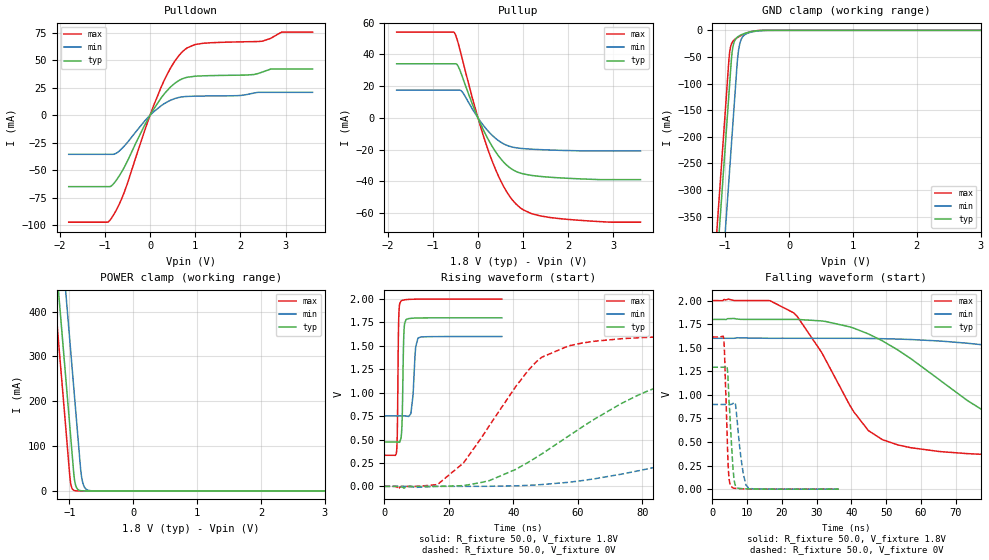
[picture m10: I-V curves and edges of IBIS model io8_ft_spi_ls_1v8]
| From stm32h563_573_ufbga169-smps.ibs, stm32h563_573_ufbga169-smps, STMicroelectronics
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[Model]   io8_ft_spi_ls_1v8
Model_type I/O
Polarity   Non-Inverting
Enable   Active-Low
| CAP_THRESHOLD on pad IOFT is "UDTCAPC" :
| Rising=20.0% of vddiom   Falling=80.0% of vddiom
| C_comp min and max val. don't necessarily correlate with the min and max pvt
| but are the smallest and greatest pad capacitance found.
| var   typ   min   max
C_comp   4.56187pF  4.45385pF  4.74999pF
|C_comp_pullup   2.85180pF  2.67180pF  2.77200pF
|C_comp_pulldown   1.71007pF  1.78205pF  1.97799pF
Vinl = 480.0mV
Vinh = 1.4V
Vmeas = 900.0mV   | Reference voltage for timing measurements
Cref  = 50.0pF   | Timing specification test load capacitance value
Rref  = 100.0MOhm   | Timing specification test load resistance value
Vref  = 900.0mV   | Timing specification test load voltage
[Model Spec]
| TIME_THRESHOLD on pin ZIV11 is "CMOS" :
| Rising=40.0% of vdd   Falling=60.0% of vdd
Vinl 703.80000mV 631.80000mV 784.80000mV
Vinh 1.06220V 937.20000mV 1.16620V
| variable   typ   min   max
[Temperature Range] 25.0 125.0 -40.0
| variable   typ   min   max
[Voltage Range] 1.8V 1.6V 2.0V
| variable   typ   min   max
[POWER Clamp Reference] 1.8V 1.6V 2.0V
| variable   typ   min   max
[GND Clamp Reference] 0V 0V 0V
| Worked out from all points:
|   slope of the pulldown table from 0 to 0.27 V, typ, clamps not added: 15.8 ohm
|   slope of the pullup table from 0 to 0.27 V, typ, clamps not added: 17.1 ohm
|   GND clamp passes 1 mA (typ) near -0.52 V on its own axis
|   POWER clamp passes 1 mA (typ) near -0.84 V on its own axis
|   rising waveform, R_fixture 50.0, V_fixture 1.8V: 20-80 % time 428ps typ, 866ps min, 322ps max; typ from 0.474 V to 1.8 V
|   falling waveform, R_fixture 50.0, V_fixture 1.8V: 20-80 % time 33.3ns typ, 83.7ns min, 16.5ns max; typ from 1.8 V to 0.474 V
|   rising waveform, R_fixture 50.0, V_fixture 0V: 20-80 % time 38.2ns typ, 81.8ns min, 20ns max; typ from 0 V to 1.29 V
|   falling waveform, R_fixture 50.0, V_fixture 0V: 20-80 % time 1.2ns typ, 1.69ns min, 842ps max; typ from 1.29 V to 0 V
[POWER Clamp]
-1.8V     1.518A     1.709A     1.407A
-1.23V    548.8mA    740.2mA    437.5mA
-1.16V    429.8mA    621.2mA    318.5mA
-1.05V    242.8mA    434.2mA    131.5mA
-980mV    123.8mA    315.2mA    17.95mA
-930mV    38.81mA    230.2mA    1.49mA
-910mV    17.82mA    196.2mA    550.8uA
-890mV    8.18mA     162.2mA    203.5uA
-810mV    363.5uA    33.6mA     3.797uA
-770mV    76.62uA    10.47mA    518.8nA
-710mV    7.417uA    1.822mA    26.38nA
3.6V      0A         0A         0A
[GND Clamp]
-1.8V     -1.581A    -1.742A    -1.516A
-1.24V    -628.8mA   -789.9mA   -564.1mA
-1.05V    -305.8mA   -466.9mA   -241.1mA
-940mV    -118.8mA   -279.9mA   -54.1mA
-930mV    -101.8mA   -262.9mA   -41.86mA
-900mV    -51.51mA   -211.9mA   -25.34mA
-880mV    -32.22mA   -177.9mA   -21mA
-810mV    -13.02mA   -59.5mA    -13.82mA
-770mV    -9.8mA     -24.99mA   -11mA
-680mV    -5.275mA   -7.288mA   -5.917mA
-400mV    -107uA     -349.1uA   -42.51uA
3.6V      5.392nA    968.2nA    261.3pA
| variable   typ   min   max
[Pullup Reference] 1.8V 1.6V 2.0V
| variable   typ   min   max
[Pulldown Reference] 0V 0V 0V
[Pullup]
-1.8V     34.12mA    17.47mA    54.1mA
-520mV    34.12mA    17.47mA    53.62mA
-450mV    33.13mA    17.47mA    48.39mA
-350mV    26.32mA    16.48mA    37.5mA
0V        9.62pA     772pA      6.41pA
300mV     -17.25mA   -10.57mA   -26.11mA
610mV     -29.08mA   -16.97mA   -45.33mA
770mV     -32.67mA   -18.47mA   -52mA
930mV     -34.74mA   -19.19mA   -56.56mA
1.18V     -36.29mA   -19.75mA   -60.37mA
1.6V      -37.46mA   -20.28mA   -62.86mA
3.6V      -38.97mA   -20.89mA   -65.81mA
[Pulldown]
-1.8V     -65.02mA   -35.56mA   -97.42mA
-940mV    -65.02mA   -35.56mA   -97.42mA
-850mV    -64.17mA   -35.56mA   -93.5mA
-570mV    -47.32mA   -28.01mA   -70.04mA
-120mV    -9.088mA   -5.278mA   -14.07mA
250mV     16.04mA    8.831mA    26.05mA
550mV     29.17mA    15.25mA    49.41mA
780mV     34.17mA    17.07mA    60.14mA
1.18V     35.97mA    17.56mA    65.65mA
2.49V     39.44mA    20.93mA    67.53mA
2.92V     42.19mA    20.93mA    75.82mA
3.6V      42.19mA    20.93mA    75.82mA
[Ramp]
dV/dt_r 775.77678mV/38.11663ns 538.06846mV/81.67179ns 968.31748mV/19.7847ns
dV/dt_f 795.72959mV/32.7099ns 504.29944mV/83.53442ns 1.00099V/15.82799ns
R_load = 50.0
| Removed startup time: 0s 0s 0s  .
| Removed end time: 36.4ns.
[Rising Waveform]
R_fixture   = 50.0
V_fixture   = 1.8V
V_fixture_min = 1.6V
V_fixture_max = 2.0V
0s        473.7mV    751.8mV    331.7mV
3.75ns    473.7mV    751.8mV    369.6mV
4ns       473.6mV    751.8mV    590.6mV
4.45ns    471.1mV    751.8mV    1.812V
5.15ns    517.7mV    751.8mV    1.979V
6.05ns    1.648V     751.8mV    1.99V
6.7ns     1.781V     751.2mV    1.994V
8.2ns     1.794V     777.2mV    1.997V
10.4ns    1.798V     1.584V     1.999V
36.4ns    1.8V       1.6V       2V
| Removed startup time: 0s 0s 0s  .
| Removed end time: 399.4ns.
[Falling Waveform]
R_fixture   = 50.0
V_fixture   = 1.8V
V_fixture_min = 1.6V
V_fixture_max = 2.0V
0s        1.8V       1.6V       2V
16.6ns    1.8V       1.6V       1.999V
23.35ns   1.8V       1.6V       1.871V
44.9ns    1.646V     1.598V     621.3mV
65.2ns    1.164V     1.571V     399.9mV
89.65ns   673.3mV    1.473V     353.8mV
122.3ns   540.5mV    1.235V     337.9mV
163.1ns   496.7mV    984.9mV    333.1mV
211.9ns   481mV      857.3mV    331.9mV
399.4ns   473.8mV    759.5mV    331.7mV
| Removed startup time: 0s 0s 0s  .
| Removed end time: 399.3ns.
[Rising Waveform]
R_fixture   = 50.0
V_fixture   = 0V
V_fixture_min = 0V
V_fixture_max = 0V
0s        134.8nV    547.2nV    93.89nV
16.7ns    -213.9uV   -97.6uV    26.34mV
24.5ns    7.415mV    -28.63uV   249.5mV
47ns      307.5mV    15.04mV    1.327V
65.2ns    719.2mV    80.86mV    1.55V
89.7ns    1.114V     248.6mV    1.6V
122.3ns   1.251V     501.7mV    1.612V
163ns     1.284V     720.1mV    1.614V
211.9ns   1.291V     837.5mV    1.614V
399.3ns   1.293V     896.8mV    1.614V
| Removed startup time: 0s 0s 0s  .
| Removed end time: 36.4ns.
[Falling Waveform]
R_fixture   = 50.0
V_fixture   = 0V
V_fixture_min = 0V
V_fixture_max = 0V
0s        1.293V     898.3mV    1.614V
3.25ns    1.293V     898.3mV    1.597V
4.15ns    1.304V     898.3mV    693mV
4.55ns    1.144V     898.2mV    252.2mV
5.25ns    639.4mV    897.8mV    37.2mV
5.95ns    220.6mV    908.8mV    13.26mV
6.6ns     41.34mV    905.9mV    8.725mV
8.6ns     5.313mV    234.7mV    3.94mV
10.4ns    2.892mV    11.51mV    2.039mV
36.4ns    369uV      126.7uV    207.2uV
